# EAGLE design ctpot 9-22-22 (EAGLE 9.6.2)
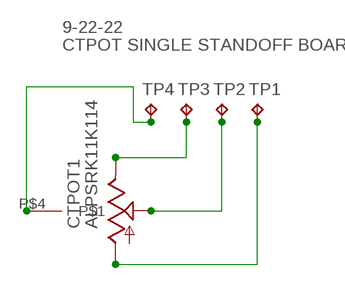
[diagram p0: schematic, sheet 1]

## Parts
CTPOT1  ALPSRK11K114  [ALPSCENTERTAP]
TP1  TPPAD1-13  [P1-13]
TP2  TPPAD1-13  [P1-13]
TP3  TPPAD1-13  [P1-13]
TP4  TPPAD1-13  [P1-13]

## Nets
N$2: CTPOT1.P$3(LOW) TP1.TP
N$3: CTPOT1.P$2(WIPER) TP2.TP
N$4: CTPOT1.P$1(HIGH) TP3.TP
N$5: CTPOT1.P$4 TP4.TP

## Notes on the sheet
- 9-22-22
- CTPOT SINGLE STANDOFF BOARD

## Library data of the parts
CTPOT1 = MusicThingModular-CL:ALPSRK11K114: ALPS Pot with center tap ground
TP1-TP4 = testpad-CL:TP: Test pad NO NAME

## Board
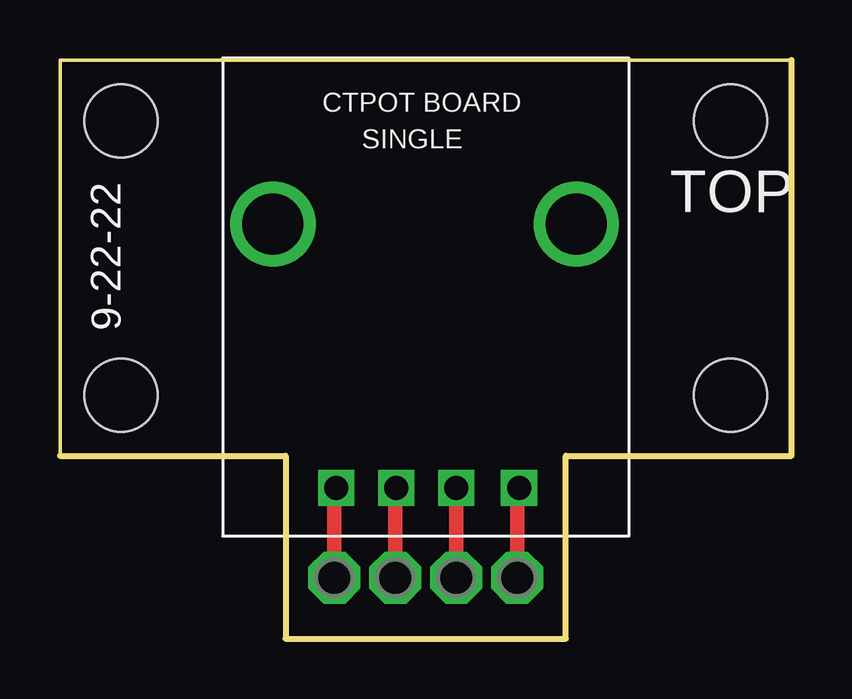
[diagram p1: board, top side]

Size 30.48 x 24.13 mm. Coordinates in mm from the lower left corner, seen from the top.
Outline: 0,24.13 0,7.62 9.4,7.62 9.4,0 21.08,0 21.08,7.62 30.48,7.62 30.48,24.13 0,24.13
Copper layers (1*16): Top 0.035mm / dielectric 1.5mm / Bottom 0.035mm
Design rules "default": minimum track width 6mil, minimum drill 0.35mm, track to track 6mil, track to pad 6mil, pad to pad 6mil, via to via 6mil, smd to smd 6mil, copper to edge 40mil, drill to drill 6mil, minimum pad ring 10mil, minimum via ring 8mil, stop-mask expansion 4mil, vias tented up to drill 0mil, thermal gap 10mil
Holes 3.05 mm at 2.54,21.59 27.94,21.59 2.54,10.16 27.94,10.16

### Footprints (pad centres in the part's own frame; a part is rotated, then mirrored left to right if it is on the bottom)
ALPSCENTERTAP = drill 1 square: P$1 10.238,3.746; P$2 12.738,3.746; P$3 15.238,3.746; P$4 17.857,3.746 | drill 2.54: P$5 7.603,14.746; P$6 20.238,14.746
P1-13 = drill 1.321 pad 2.159 octagon: TP 0,0

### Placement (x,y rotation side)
CTPOT1  1.27,2.54 0 top
TP1  16.51,2.54 0 top
TP2  13.97,2.54 180 top
TP3  11.43,2.54 0 top
TP4  19.05,2.54 0 top

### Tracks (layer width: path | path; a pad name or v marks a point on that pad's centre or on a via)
N$2
  Top 0.152: CTPOT1.P$3
  Top 0.61: TP1.TP CTPOT1.P$3
N$3
  Top 0.152: 13.97,6.25 CTPOT1.P$2
  Top 0.61: TP2.TP 13.97,6.25
N$4
  Top 0.152: 11.43,6.21 CTPOT1.P$1
  Top 0.61: TP3.TP 11.43,6.21
N$5
  Top 0.152: 19.05,6.21 CTPOT1.P$4
  Top 0.61: TP4.TP 19.05,6.21

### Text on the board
tNames: CTPOT BOARD | SINGLE | 9-22-22 | TOP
